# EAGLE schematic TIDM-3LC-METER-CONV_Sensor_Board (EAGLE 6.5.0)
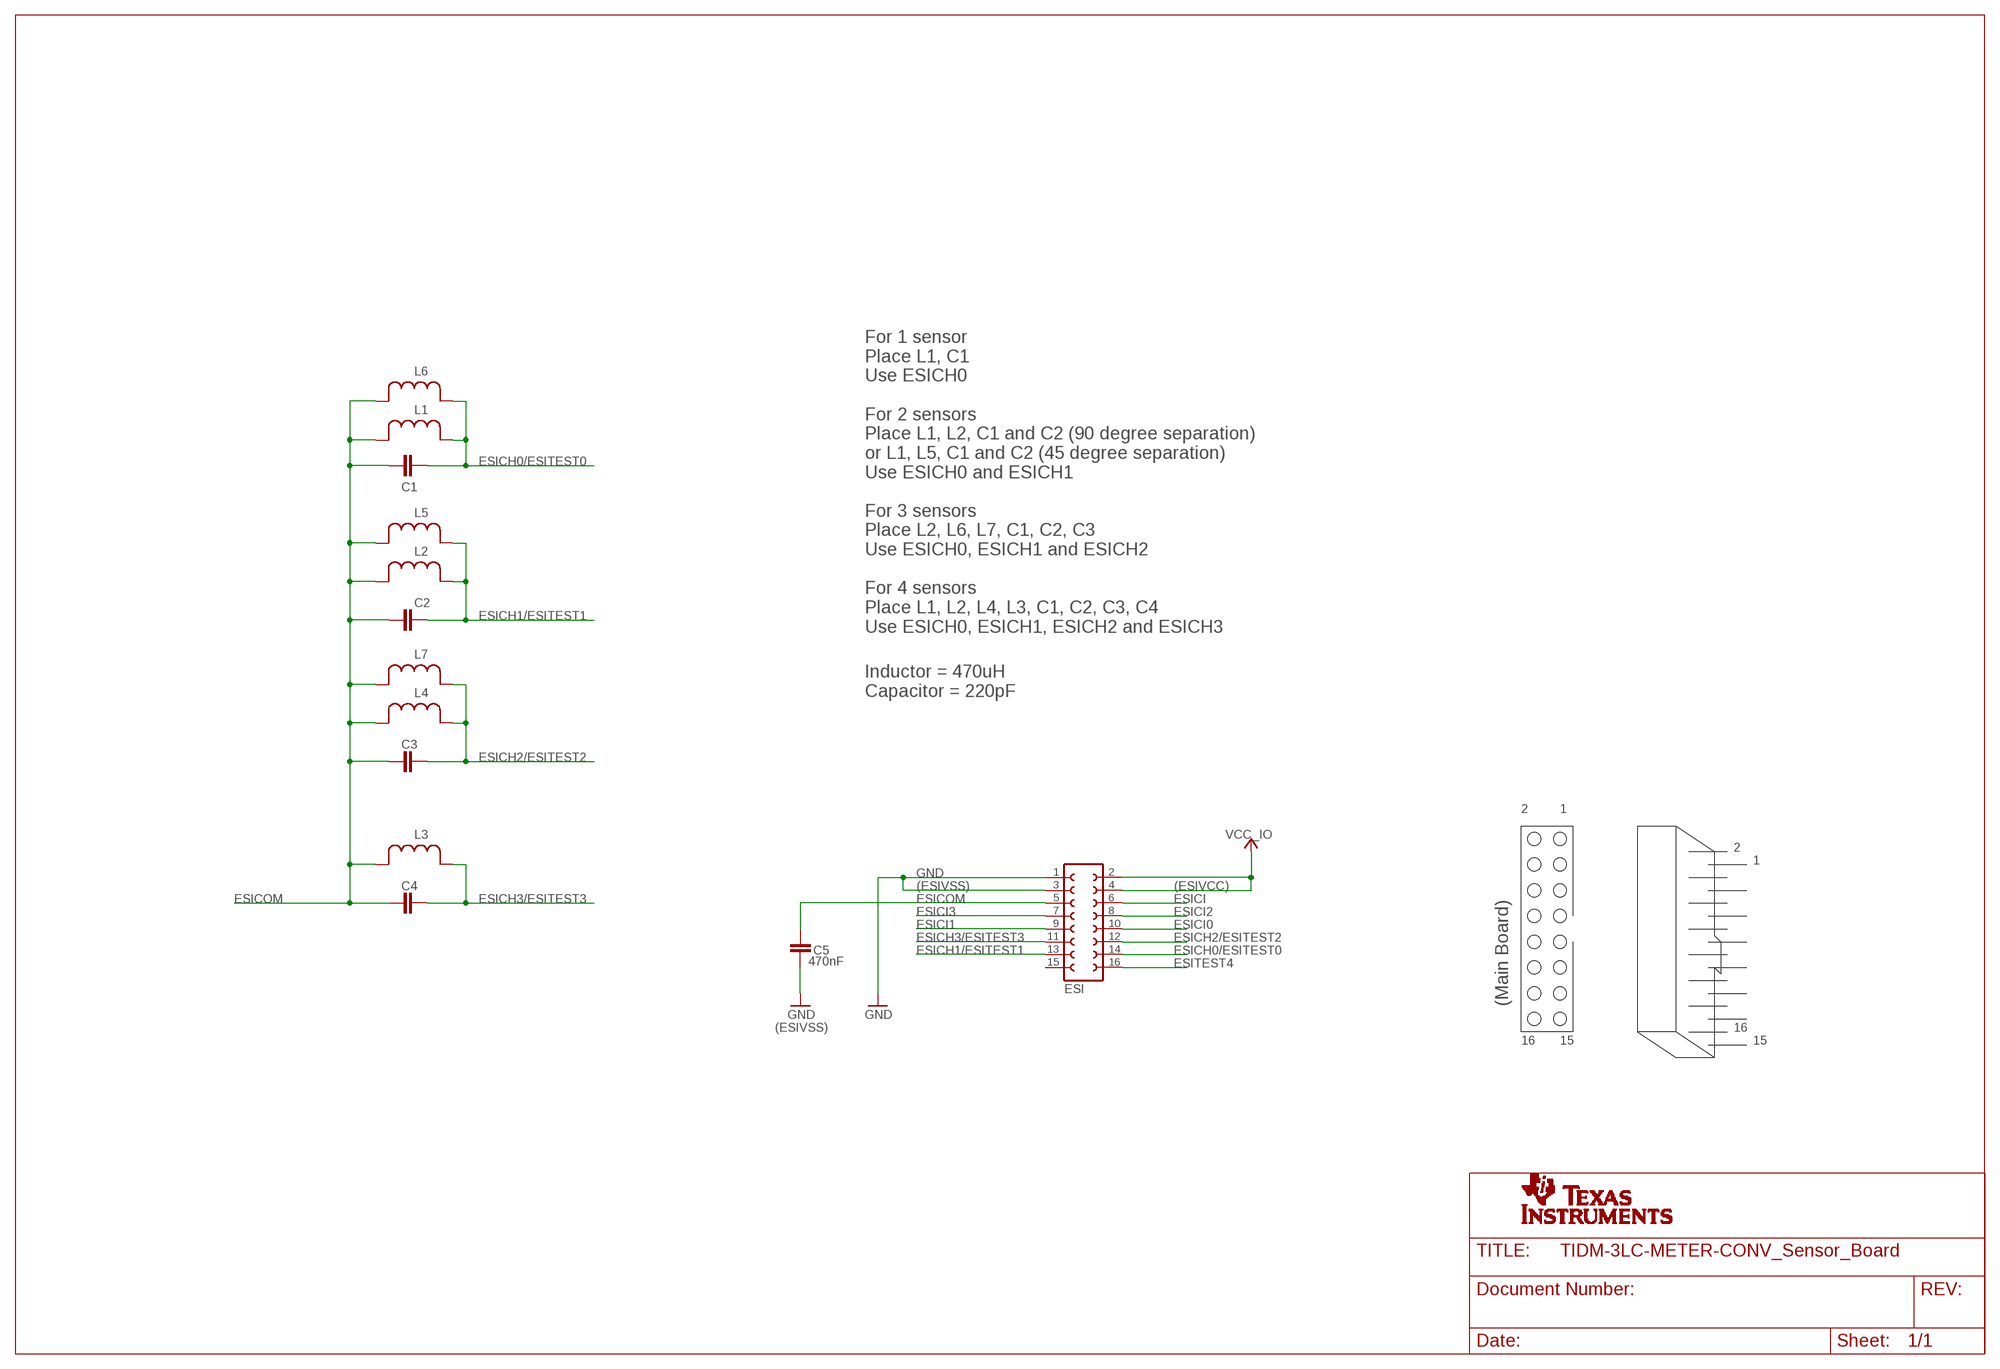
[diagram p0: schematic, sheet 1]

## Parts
C1  220pF  C-EUC0402  [C0402]
C2  220pF  C-EUC0402  [C0402]
C3  DNP  C-EUC0402  [C0402]
C4  DNP  C-EUC0402  [C0402]
C5  470nF  C-EUC0603  [C0603]
ESI  FE08-2  [FE08-2]
L1  470uH  LR_SENSOR  [0204/7]
L2  470uH  LR_SENSOR  [0204/7]
L3  DNP  LR_SENSOR  [0204/7]
L4  DNP  LR_SENSOR  [0204/7]
L5  DNP  LR_SENSOR  [0204/7]
L6  DNP  LR_SENSOR  [0204/7]
L7  DNP  LR_SENSOR  [0204/7]
U$1  TI-LOGO-SMALL  [TI-LOGO-4]

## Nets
ESICH0/ESITEST0: C1.2 ESI.14 L1.2 L6.2
ESICH1/ESITEST1: C2.2 ESI.13 L2.2 L5.2
ESICH2/ESITEST2: C3.2 ESI.12 L4.2 L7.2
ESICH3/ESITEST3: C4.2 ESI.11 L3.2
ESICI: ESI.6
ESICI0: ESI.10
ESICI1: ESI.9
ESICI2: ESI.8
ESICI3: ESI.7
ESICOM: C1.1 C2.1 C3.1 C4.1 C5.1 ESI.5 L1.1 L2.1 L3.1 L4.1 L5.1 L6.1 L7.1
ESITEST4: ESI.16
GND: C5.2 ESI.1 ESI.3
VCC_IO: ESI.2 ESI.4
Unconnected: ESI.15

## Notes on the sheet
- For 1 sensor
  Place L1, C1
  Use ESICH0
  
  For 2 sensors
  Place L1, L2, C1 and C2 (90 degree separation)
  or L1, L5, C1 and C2 (45 degree separation)
  Use ESICH0 and ESICH1
  
  For 3 sensors
  Place L2, L6, L7, C1, C2, C3
  Use ESICH0, ESICH1 and ESICH2
  
  For 4 sensors
  Place L1, L2, L4, L3, C1, C2, C3, C4
  Use ESICH0, ESICH1, ESICH2 and ESICH3
- Inductor = 470uH
  Capacitor = 220pF
- 2 | 1
- 2
- 1
- (ESIVSS) | (ESIVCC)
- (Main Board)
- (ESIVSS) | 16
- 16 | 15 | 15

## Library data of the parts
C1-C5 = rcl:C-EU: CAPACITOR, European symbol
ESI = con-lsta:FE08-2: FEMALE HEADER; OC_FARNELL: unknown; OC_NEWARK: unknown
L1-L7 = Sensor LR:LR_SENSOR
U$1 = texas-logo:TI-LOGO: Full TI logo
